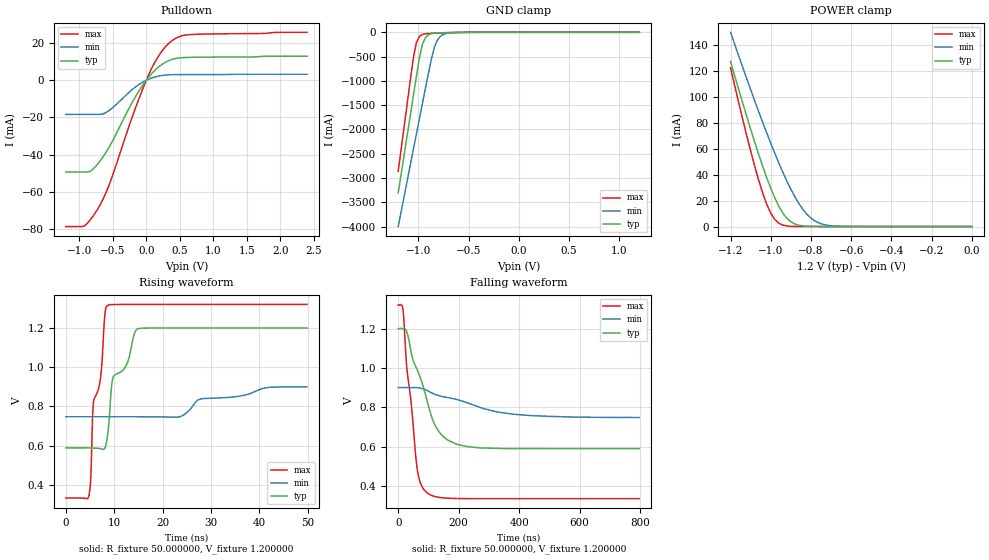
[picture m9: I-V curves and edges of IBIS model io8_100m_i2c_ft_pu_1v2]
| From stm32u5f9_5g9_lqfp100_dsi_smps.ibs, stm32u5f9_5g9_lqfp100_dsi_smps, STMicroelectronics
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|   Model io8_100m_i2c_ft_pu_1v2
[Model]  io8_100m_i2c_ft_pu_1v2
Model_type I/O_open_drain
Polarity   Non-Inverting
Enable   Active-Low
Vinl =   0.360000V
Vinh =   0.840000V
Vmeas =  0.600000V
Cref =   50.000000pF
Rref =   100.000000M
Vref =   0.600000V
C_comp   2.954600pF   2.884400pF   3.002700pF
[Temperature Range]   25.000000   0.140000k   -40.000000
[Pullup Reference]   1.200000V   0.900000V   1.320000V
[Pulldown Reference]   0.0V   0.0V   0.0V
[POWER Clamp Reference]   1.200000V   0.900000V   1.320000V
[GND Clamp Reference]   0.0V   0.0V   0.0V
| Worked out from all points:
|   slope of the pulldown table from 0 to 0.18 V, typ, clamps not added: 25.7 ohm
|   GND clamp passes 1 mA (typ) near -0.51 V on its own axis
|   POWER clamp passes 1 mA (typ) near -0.86 V on its own axis
|   rising waveform, R_fixture 50.000000, V_fixture 1.200000: 20-80 % time 4.46ns typ, 13ns min, 2.41ns max; typ from 0.589 V to 1.2 V
|   falling waveform, R_fixture 50.000000, V_fixture 1.200000: 20-80 % time 78ns typ, 207ns min, 36ns max; typ from 1.2 V to 0.589 V
[Pulldown]
|Voltage   I(typ)   I(min)   I(max)
-1.2V     -49.24mA   -18.34mA   -78.58mA
-920mV    -49.24mA   -18.34mA   -78.22mA
-840mV    -48.98mA   -18.34mA   -75.14mA
-720mV    -44.76mA   -18.34mA   -68.87mA
-560mV    -36.26mA   -16.38mA   -56.73mA
-200mV    -11.29mA   -4.684mA   -18.8mA
0V        0A         0A         0A
160mV     6.399mA    2.052mA    11.64mA
360mV     10.86mA    2.957mA    20.57mA
480mV     11.93mA    3.021mA    23.25mA
640mV     12.29mA    3.041mA    24.48mA
2.4V      12.9mA     3.221mA    25.75mA
[GND_clamp]
|Voltage   I(typ)   I(min)   I(max)
-1.2V     -3.305A    -3.998A    -2.862A
-1.05V    -1.316A    -2.418A    -539.3mA
-1.02V    -921mA     -2.103A    -218.8mA
-990mV    -539.5mA   -1.788A    -87.43mA
-960mV    -252.1mA   -1.474A    -44.36mA
-930mV    -110.5mA   -1.16A     -30.32mA
-870mV    -28.03mA   -549.1mA   -21.09mA
-840mV    -18.43mA   -305.6mA   -18.27mA
-810mV    -13.9mA    -159.7mA   -15.73mA
-780mV    -11.23mA   -82.35mA   -13.37mA
-600mV    -2.976mA   -4.272mA   -3.058mA
1.2V      0A         14.74nA    0A
[POWER_clamp]
|Voltage   I(typ)   I(min)   I(max)
-1.2V     127mA      149.4mA    122.2mA
-1.12V    84.98mA    114mA      70.29mA
-1.06V    55.52mA    88.42mA    35.69mA
-1.02V    37.64mA    72.04mA    17.19mA
-1V       29.52mA    64.13mA    10.33mA
-960mV    15.7mA     48.99mA    2.596mA
-900mV    3.636mA    28.77mA    207.8uA
-840mV    502.9uA    13.24mA    43.42uA
-800mV    129uA      6.535mA    43.42uA
-740mV    25.7uA     1.726mA    43.42uA
-620mV    25.17uA    82.33uA    35.63uA
0V        0A         17.33nA    0A
[Ramp]
| variable   typ   min   max
dV/dt_r  0.36637/4.45106n   91.26600m/13.03316n 0.59131/2.40467n
dV/dt_f  0.36649/77.97422n   91.18200m/0.20660u  0.59143/35.98370n
R_load = 50.000000
[Rising Waveform]
R_fixture= 50.000000
V_fixture= 1.200000
V_fixture_min= 0.900000
V_fixture_max= 1.320000
|time   V(typ)   V(min)   V(max)
0s        589.2mV    747.7mV    334.3mV
4.805ns   589.2mV    747.7mV    351.4mV
5.105ns   588.9mV    747.7mV    416mV
5.706ns   588.3mV    747.7mV    820.9mV
7.107ns   585.6mV    747.7mV    936mV
8.008ns   585.6mV    747.7mV    1.255V
8.509ns   633.8mV    747.7mV    1.312V
9.71ns    944.9mV    747.7mV    1.319V
14.71ns   1.194V     747.7mV    1.32V
49.85ns   1.2V       900mV      1.32V
[Falling Waveform]
R_fixture= 50.000000
V_fixture= 1.200000
V_fixture_min= 0.900000
V_fixture_max= 1.320000
|time   V(typ)   V(min)   V(max)
0s        1.2V       900mV      1.32V
16.02ns   1.2V       900.5mV    1.295V
28.83ns   1.183V     900.3mV    996.3mV
43.24ns   1.076V     900mV      814.9mV
64.06ns   986.4mV    899.4mV    473.5mV
94.49ns   838.7mV    886.2mV    365.4mV
129.7ns   687.1mV    861.2mV    342.4mV
193.8ns   611.2mV    839.1mV    335.2mV
382.8ns   589.3mV    764.2mV    334.3mV
797.6ns   589.2mV    747.7mV    334.3mV
